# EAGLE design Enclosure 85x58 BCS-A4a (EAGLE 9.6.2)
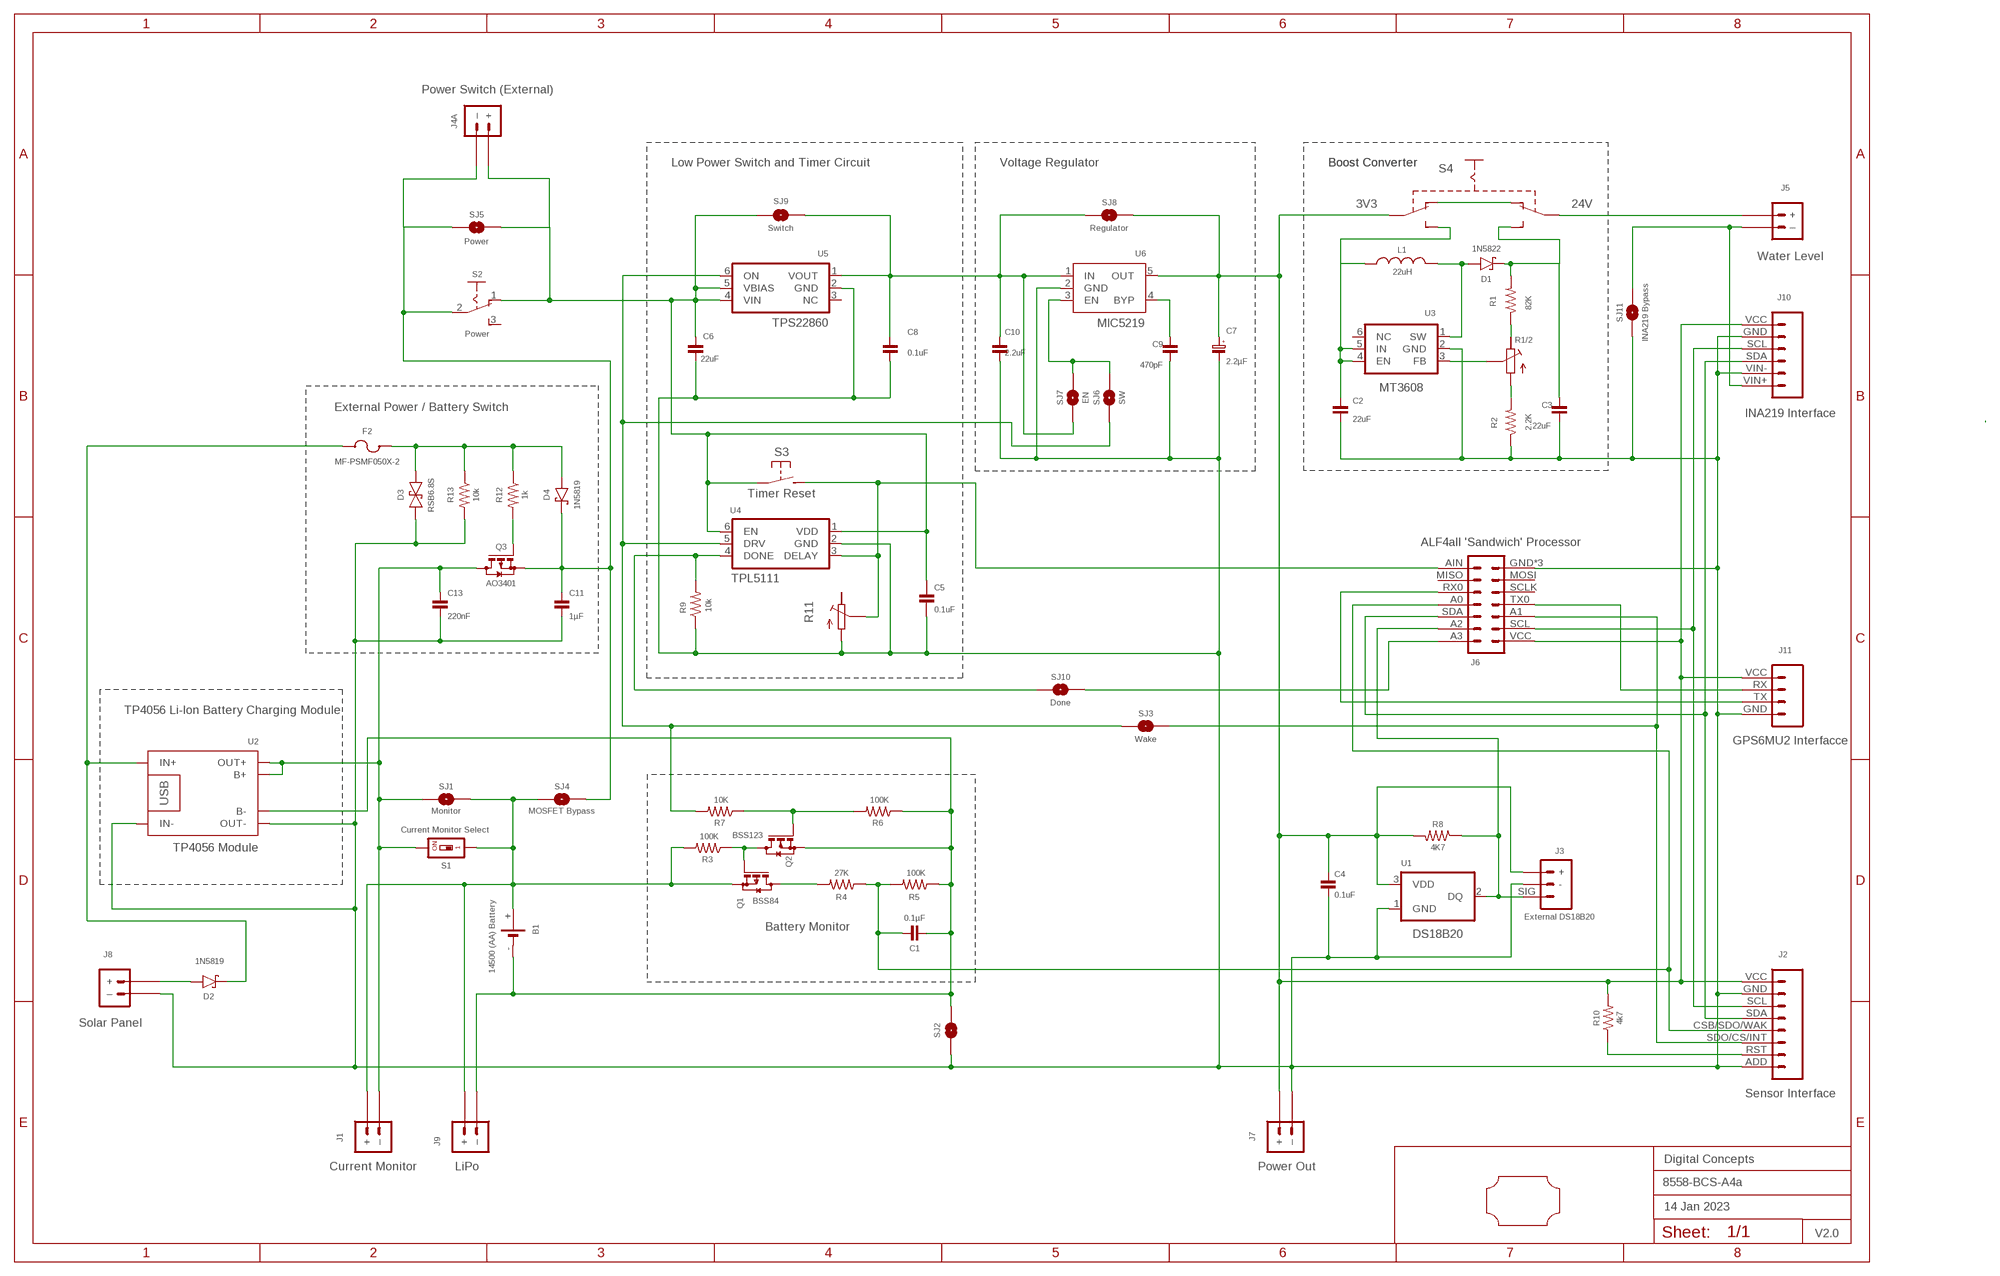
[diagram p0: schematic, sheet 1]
FRAME2 (A3L-LOC): DATE: 14 Jan 2023; OWNER: Digital Concepts; TITLE: 8558-BCS-A4a; VERSION: V2.0

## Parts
B1  14500 (AA) Battery  BATTERY-HOLDER-14500(AA)  [BATTERY-14500]
C1  0.1µF  CAPACITOR-0805  [C0805]
C2  22uF  CAPACITOR-1206  [C1206]
C3  22uF  CAPACITOR-1206  [C1206]
C4  0.1uF  CAPACITOR-0805  [C0805]
C5  0.1uF  CAPACITOR  [C0805@1]
C6  22uF  CAPACITOR-1206  [C1206]
C7  2.2µF  CAPACITOR-1206-TANTALUM  [C1206-POLARISED]
C8  0.1uF  CAPACITOR-0805  [C0805]
C9  470pF  CAPACITOR-0805  [C0805]
C10  2.2uF  CAPACITOR-0805  [C0805]
C11  1µF  CAPACITOR-0805  [C0805]
C13  220nF  CAPACITOR-0805  [C0805]
D1  1N5822  DIODE-SCHOTTKY-1N5822  [DIODE_SMB]
D2  1N5819  1N5819-SOD-123  [SOD-123]
D3  RSB6.8S  DIODE-SCHOTTKY-BIDIRECTIONAL  [VMD2]
D4  1N5819  DIODE-SCHOTTKY-1N5819  [SOD-123]
F2  MF-PSMF050X-2  [F0805]
J1  Current Monitor  JST-PH2.0-2-H-POWER  [JST-PH2.0-2-HORIZONTAL-POWER]
J2  Sensor Interface  HEADER-1X8-SENSOR  [CONN_08-SENSOR]
J3  External DS18B20  JST-PH2.0-3-VERTICAL-SIG  [JST-PH2.0-3-VERTICAL-SIG]
J4A  Power Switch (External)  JST-PH2.0-2-DUAL-POWER"  [JST-PH2.0-2-DUAL-POWER]
J5  Water Level  JST-PH2.0-2-VERTICAL-POWER  [JST-PH2.0-2-VERTICAL-POWER]
J6  ALF4all 'Sandwich' Processor  ALF4ALL-PROCESSOR-BOARD  [ALF4ALL-PROCESSOR-BOARD]
J7  Power Out  JST-GH1.25-2-VERTICAL-POWER  [JST-GH1.25-2-VERTICAL-POWER]
J8  Solar Panel  JST-PH2.0-2-VERTICAL-POWER  [JST-PH2.0-2-VERTICAL-POWER]
J9  LiPo  JST-PH2.0-2-H-POWER  [JST-PH2.0-2-HORIZONTAL-POWER]
J10  INA219 Interface  INA219-I2C-MODULE  [CONN_06-INA219]
J11  GPS6MU2 Interfacce  HEADER-1X4-GPS  [CONN_04-GPS]
L1  22uH  INDUCTOR-CDRH104R/6D28L5038P  [CDRH104R+6D28]
Q1  BSS84  [SOT23]
Q2  BSS123  [SOT23]
Q3  AO3401  MOSFET-AO3401  [SOT-23]
R1  82K  RESISTORR0805  [R0805]
R1/2  RESISTOR-TRIMM-BAOTER-HORIZONTAL  [RTRIM64P]
R2  2.2K  RESISTOR-VIA-1  [R0805-VIA-1]
R3  100K  RESISTORR0805  [R0805]
R4  27K  RESISTORR0805  [R0805]
R5  100K  RESISTORR0805  [R0805]
R6  100K  RESISTORR0805  [R0805]
R7  10K  RESISTORR0805  [R0805]
R8  4K7  RESISTORR0805  [R0805]
R9  10k  RESISTOR-VIA-2  [R0805-VIA-2]
R10  4k7  RESISTORR0805  [R0805]
R11  RESISTOR-TRIMM-BAOTER-HORIZONTAL  [RTRIM64P]
R12  1k  RESISTORR0805  [R0805]
R13  10k  RESISTORR0805  [R0805]
S1  Current Monitor Select  SWITCH-DIP-SWS001-VIA-1  [SMD-001-VIA-1]
S2  Power  SWITCH-SLIDE-SPDT  [SWITCH-SLIDE-SPDT]
S3  Timer Reset  SWITCH-MOMENTARY-2-PIN  [SWITCH-2-PAD]
S4  SWITCH-SLIDE-DPDT-PTH-S  [SWITCH-DPDT-PTH]
SJ1  Monitor  SJ  [SJ]
SJ2  Charge  SJ-V-1  [SJ-VIA-1]
SJ3  Wake  SJ-V-1  [SJ-VIA-1]
SJ4  MOSFET Bypass  SJ  [SJ]
SJ5  Power  SJ-V-1  [SJ-VIA-1]
SJ6  SW  SJ  [SJ]
SJ7  EN  SJ  [SJ]
SJ8  Regulator  SJ  [SJ]
SJ9  Switch  SJ  [SJ]
SJ10  Done  SJ-V-2  [SJ-VIA-2]
SJ11  INA219 Bypass  SJ  [SJ]
U1  DS18B20  [TO-92]
U2  TP4056 Module  BATTERY-CHARGER-LI-PROT  [BATTERY-CHARGER-LI-PROT]
U3  MT3608  [SOT-23-6]
U4  TPL5111  TPL5111DDCR  [SOT-23-6]
U5  TPS22860  [SOT-23-6]
U6  MIC5219  MIC5219XX  [SOT-23-5]
U$1  PCB-OUTLINE-CA-85X58  [PROTO-28X18-OUTLINE-CA]

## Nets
GND: C2.2 C3.2 C4.2 C5.1 C6.2 C7.2(-) C8.1 C9.2 C10.1 C11.2 C13.2 D3.P$2 J2.ADD J2.GND J3.- J6.GND J6.GND@TL J6.GND@TR J7.-(–) J8.-(–) J10.GND J10.VIN- J11.GND R2.1 R2.1@VIA R9.1 R11.1(A) R13.2 SJ2.1 SJ2.1@V SJ11.1 U1.1(GND) U2.IN- U2.OUT- U3.2(GND) U4.2(GND) U5.2(GND) U6.2(GND)
N$1: D2.A J8.+
N$2: C11.1 D4.C J4A.-(–) Q3.2(S) S2.2(P) SJ4.2 SJ5.2
N$3: B1.+ J1.+ J9.+ Q1.2(S) R3.2 S1.1 S1.1@VIA SJ1.2 SJ4.1
N$5: D2.C F2.1 U2.IN+
N$6: D1.A L1.2 U3.1(SW)
N$7: C9.1 U6.4(BYP)
N$8: J2.SCL J6.SCL J10.SCL
N$9: J2.RST R10.1
N$10: C1.1 J2.CSB/SDO/WAK J6.A0 R4.1 R5.2
N$11: J2.SDA J6.SDA J10.SDA
N$13: J3.SIG J6.A2 R8.1 U1.2(DQ)
N$14: J6.TX0 J11.RX
N$15: J5.-(–) J10.VIN+ SJ11.2
N$16: J6.RX0 J11.TX
N$18: C13.1 J1.-(–) Q3.3(D) S1.2 SJ1.1 U2.B+ U2.OUT+
N$19: SJ6.2 SJ7.2 U6.3(EN)
N$20: C8.2 C10.2 SJ7.1 SJ8.1 SJ9.1 U5.1(VOUT) U6.1(IN)
N$22: J6.A3 SJ10.1
N$23: Q1.3(D) R4.2
N$24: C2.1 L1.1 U3.4(EN) U3.5(IN)
N$25: J6.AIN R11.2(S) S3.P$2(S) U4.3(DELAY)
N$27: C5.2 C6.1 J4A.+ S2.1(O) S3.P$1(P) SJ5.1 SJ5.1@V SJ9.2 U4.1(VDD) U4.6(EN) U5.4(VIN) U5.5(VBIAS)
N$28: R7.2 SJ3.2 SJ6.1 U4.5(DRV) U5.6(ON)
N$29: R9.2 R9.2@VIA SJ10.2 SJ10.2@V U4.4(DONE)
N$30: J2.SDO/CS/INT J6.A1 SJ3.1 SJ3.1@V
N$31: C3.1 D1.C R1.2
N$32: R1.1 R1/2.3(E)
N$33: R1/2.2(S) U3.3(FB)
N$34: R1/2.1(A) R2.2
N$35: Q1.1(G) Q2.3(D) R3.1
N$36: S4.P$6(S2)
N$37: Q2.1(G) R6.2 R7.1
N$38: B1.- C1.2 J9.-(–) Q2.2(S) R5.1 R6.1 SJ2.2 U2.B-
N$39: S4.P$1(O1) S4.P$4(O2)
N$41: S4.P$3(S1)
N$42: J5.+ S4.P$5(P2)
N$43: Q3.1(G) R12.2
N$44: D3.P$1 D4.A F2.2 R12.1 R13.1
VCC: C4.1 C7.1(+) J2.VCC J3.+ J6.VCC J7.+ J10.VCC J11.VCC R8.2 R10.2 S4.P$2(P1) SJ8.2 U1.3(VDD) U6.5(OUT)
Unconnected: J6.MISO J6.MOSI J6.SCLK R11.3(E) S2.3(S) U3.6(NC) U5.3(NC)

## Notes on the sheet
- Low Power Switch and Timer Circuit | Voltage Regulator | Boost Converter | Boost Converter
- 3V3 | 24V
- External Power / Battery Switch
- TP4056 Li-Ion Battery Charging Module
- Battery Monitor

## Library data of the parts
B1 = digitalconcepts:BATTERY-HOLDER-14500(AA): 14500 (AA) battery holder
C1 C4 C8-C11 C13 = digitalconcepts:CAPACITOR-0805: 0805 Capacitor
C2 C3 C6 = digitalconcepts:CAPACITOR-1206: 1206 Capacitor
C5 = digitalconcepts:CAPACITOR: 0805 Capacitor
C7 = digitalconcepts:CAPACITOR-1206-TANTALUM: Capacitor 1206 Tantalum
D1 = digitalconcepts:DIODE-SCHOTTKY-1N5822: 1N5822 Schottky Diode SMB
D2 = digitalconcepts:1N5819-SOD-123: 1N5819 Schottky Diode SOD-123
D3 = digitalconcepts:DIODE-SCHOTTKY-BIDIRECTIONAL: Schottky Bidirectional Diode
D4 = digitalconcepts:DIODE-SCHOTTKY-1N5819: 1N5819 Schottky Diode SOD-123
F2 = digitalconcepts:MF-PSMF050X-2: PTC Resettable Fuse
J1 J9 = digitalconcepts:JST-PH2.0-2-H-POWER: JST PH2.0 2P Right Angle Connector with power pin labelling
J2 = digitalconcepts:HEADER-1X8-SENSOR: IoT Sensors 1x8 Pin Header for 'Sandwich' IoT Sensors
J3 = digitalconcepts:JST-PH2.0-3-VERTICAL-SIG: PH2.0 3P Vertical Connector (Sig)
J4A = digitalconcepts:JST-PH2.0-2-DUAL-POWER: PH2.0 2P PTH Dual-Side Connector (Power); PROD_ID: CONN-09863; SKU: PRT-09914
J5 J8 = digitalconcepts:JST-PH2.0-2-VERTICAL-POWER: JST PH2.0 2P PTH Connector (Power)
J6 = digitalconcepts:ALF4ALL-PROCESSOR-BOARD: ALF4all 'Sandwixh' Processor 2x7 Pin Header and earthed 1x1 locator pins for ALF4all 'Sandwich' Processor/RFM95W PCBs
J7 = digitalconcepts:JST-GH1.25-2-VERTICAL-POWER: JST GH1.25 2P PTH Connector (Power)
J10 = digitalconcepts:INA219-I2C-MODULE: INA219 I2C Module
J11 = digitalconcepts:HEADER-1X4-GPS: NEO GPS 4-Pin Header
L1 = digitalconcepts:INDUCTOR-CDRH104R/6D28: Inductor; SPICEPREFIX: L
Q1 = digitalconcepts:BSS84: P-CHANNEL MOS FET
Q2 = digitalconcepts:BSS123: N-CHANNEL MOS FET
Q3 = digitalconcepts:MOSFET-AO3401: AO3401 P-Channel MOSFET
R1 R3-R8 R10 R12 R13 = digitalconcepts:RESISTOR: Resistor; SPICEPREFIX: R
R1/2 R11 = digitalconcepts:RESISTOR-TRIMM-BAOTER-HORIZONTAL: Trimm Resistor - Horizontal BAOTER
R2 = digitalconcepts:RESISTOR-VIA-1: Resistor with via on Pad 1
R9 = digitalconcepts:RESISTOR-VIA-2: Resistor with via on Pad 2
S1 = digitalconcepts:SWITCH-DIP-SWS001-VIA-1: SMD Dip Switch 1 pol.
S2 = digitalconcepts:SWITCH-SLIDE-SPDT: Mini Sliding Switch SPDT
S3 = digitalconcepts:SWITCH-MOMENTARY-2-PIN: 2 Pin Momentary Switch
S4 = digitalconcepts:SWITCH-SLIDE-DPDT-PTH-S: Switch DPDT PTH-S
SJ1 SJ4 SJ6-SJ9 SJ11 = digitalconcepts:SJ: Solder Jumper
SJ2 SJ3 SJ5 = digitalconcepts:SJ-V-1: Solder Jumper with single Pad Via
SJ10 = digitalconcepts:SJ-V-2: Solder Jumper with Pad Vias
U1 = digitalconcepts:DS18B20: Digital Thermometer -55C-125C TO92-3; AVAILABILITY: Bad; DESCRIPTION: Temperature Sensor Digital, Local -55°C ~ 125°C 12 b 8-uMAX; MF: Maxim Integrated; MP: DS18B20; PACKAGE: TO-92 Maxim Integrated; PRICE: None
U2 = digitalconcepts:BATTERY-CHARGER-LI-PROT: TP4056 Li Battery Charger module with PCB (rather than module) footprint
U3 = digitalconcepts:MT3608: MT3608 DC-DC Step-Up Voltage Converter
U4 = digitalconcepts:TPL5111DDCR: TPL5111 Nano-Power System Timer
U5 = digitalconcepts:TPS22860: Texas Instruments TPS22860 Ultra-Low Leakage Load Switch
U6 = digitalconcepts:MIC5219XX: VOLTAGE REGULATOR; OC_FARNELL: unknown; OC_NEWARK: unknown
U$1 = digitalconcepts:PCB-OUTLINE-CA-85X58: PCB outline with cut-out for 85 x 58 enclosure

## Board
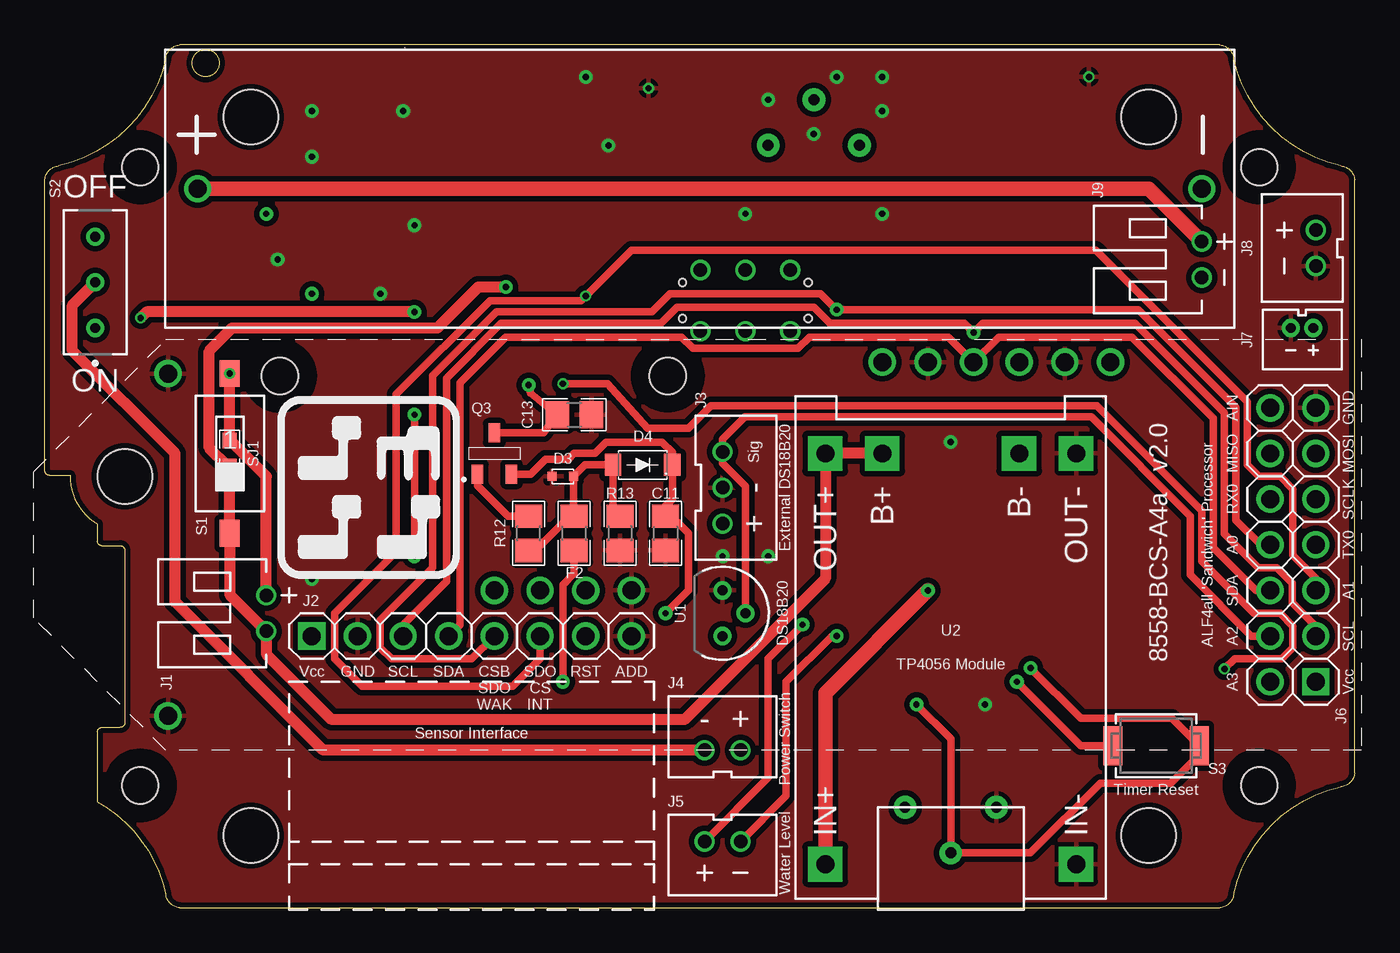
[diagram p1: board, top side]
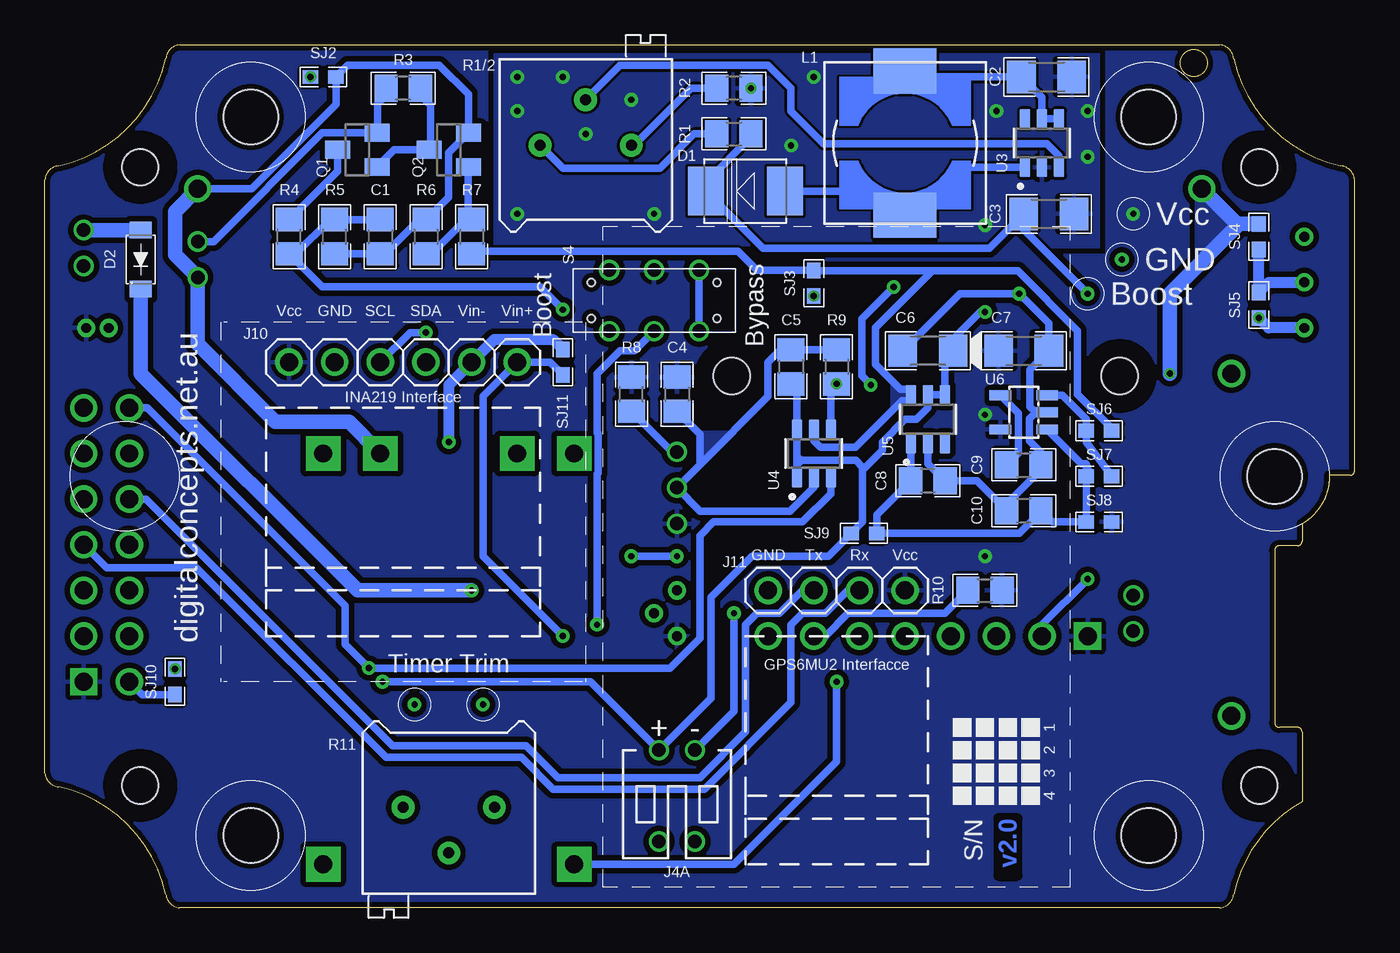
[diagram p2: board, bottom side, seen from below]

Size 72.9 x 48.01 mm. Coordinates in mm from the lower left corner, seen from the top.
Copper layers (1*16): Top 0.035mm / dielectric 1.5mm / Bottom 0.035mm
Design rules "default *": minimum track width 6mil, minimum drill 0.35mm, track to track 6mil, track to pad 6mil, pad to pad 6mil, via to via 6mil, smd to smd 6mil, copper to edge 6mil, drill to drill 6mil, minimum pad ring 1mil, minimum via ring 8mil, stop-mask expansion 4mil, vias tented up to drill 0mil, thermal gap 10mil
Holes 2.03 mm at 13.08,29.59 34.67,29.59

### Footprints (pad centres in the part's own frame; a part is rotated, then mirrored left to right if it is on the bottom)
BATTERY-14500 = drill 1: + -27.94,0; - 27.94,0
C0805 = smd 1.3 x 1.5: 1 -0.95,0; 2 0.95,0
C1206 = smd 1.6 x 1.8: 1 -1.4,0; 2 1.4,0
C0805@1 = smd 1.3 x 1.5: 1 -0.95,0; 2 0.95,0
C1206-POLARISED = smd 1.6 x 1.8: 1 -1.4,0; 2 1.4,0
DIODE_SMB = smd 2 x 2.7: A 2.2,0; C -2.2,0
SOD-123 = smd 0.91 x 1.22: A -1.65,0; C 1.65,0
VMD2 = smd 0.5 x 0.5: P$1 -0.6,0; P$2 0.6,0
F0805 = smd 1.3 x 1.5: 1 -0.95,0; 2 0.95,0
JST-PH2.0-2-HORIZONTAL-POWER = drill 0.75: + 1,0; - -1,0
CONN_08-SENSOR = drill 1 pad 1.524: ADD 17.78,0; CSB/SDO/WAK 10.16,0; GND 2.54,0; RST 15.24,0; SCL 5.08,0; SDA 7.62,0; SDO/CS/INT 12.7,0 | drill 1 pad 1.524 square: VCC 0,0
JST-PH2.0-3-VERTICAL-SIG = drill 0.75: + -2,0; - 0,0; SIG 2,0
JST-PH2.0-2-DUAL-POWER = drill 0.75: + 1,0; - -1,0
JST-PH2.0-2-VERTICAL-POWER = drill 0.75: + -1,0; - 1,0
ALF4ALL-PROCESSOR-BOARD = drill 1 pad 1.524: A0 7.62,2.54; A1 5.08,0; A2 2.54,2.54; A3 0,2.54; AIN 15.24,2.54; GND 15.24,0; GND@TL -1.905,63.881; GND@TR 17.145,63.881; MISO 12.7,2.54; MOSI 12.7,0; RX0 10.16,2.54; SCL 2.54,0; SCLK 10.16,0; SDA 5.08,2.54; TX0 7.62,0 | drill 1 pad 1.524 square: VCC 0,0
JST-GH1.25-2-VERTICAL-POWER = drill 0.55 pad 1.016: + 0.625,0; - -0.625,0
CONN_06-INA219 = drill 1 pad 1.524: GND 2.54,0; SCL 5.08,0; SDA 7.62,0; VCC 0,0; VIN+ 12.7,0; VIN- 10.16,0
CONN_04-GPS = drill 1 pad 1.524: GND 0,0; RX 5.08,0; TX 2.54,0; VCC 7.62,0
CDRH104R+6D28 = smd 2.5 x 3.5: 1 -4,0; 2 4,0
SOT23 = smd 1 x 1.4: 1 -0.95,-1.1; 2 0.95,-1.1; 3 0,1.1
SOT-23 = smd 0.65 x 1.05: 1 -0.95,-1.15; 2 0.95,-1.15; 3 0,1.15
R0805 = smd 1.3 x 1.5: 1 -0.95,0; 2 0.95,0
RTRIM64P = drill 0.61 pad 1.27: 1 0,-2.54; 2 2.54,0; 3 0,2.54
R0805-VIA-1 = smd 1.3 x 1.5: 1 -0.95,0; 2 0.95,0 | drill 0.35 pad 0.61: 1@VIA -0.95,0
R0805-VIA-2 = smd 1.3 x 1.5: 1 -0.95,0; 2 0.95,0 | drill 0.35 pad 0.61: 2@VIA 0.95,0
SMD-001-VIA-1 = smd 1.1 x 1.5: 1 0,-4.45; 2 0,4.45 | drill 0.35 pad 0.61: 1@VIA 0,-4.45
SWITCH-SLIDE-SPDT = drill 0.55 pad 1.016: 1 -2.54,0; 2 0,0; 3 2.54,0
SWITCH-2-PAD = smd 1.067 x 2.184: P$1 -2.4,0; P$2 2.4,0
SWITCH-DPDT-PTH = drill 0.75: P$1 -1.7,2.5; P$2 -1.7,0; P$3 -1.7,-2.5; P$4 1.7,2.5; P$5 1.7,0; P$6 1.7,-2.5 | hole 0.42: 1,3.5; -1,3.5; 1,-3.5; -1,-3.5
SJ = smd 0.864 x 0.762: 1 -0.711,0; 2 0.711,0
SJ-VIA-1 = smd 0.864 x 0.762: 1 -0.711,0; 2 0.711,0 | drill 0.35 pad 0.61: 1@V -0.711,0
SJ-VIA-2 = smd 0.864 x 0.762: 1 -0.711,0; 2 0.711,0 | drill 0.35 pad 0.61: 2@V 0.711,0
TO-92 = drill 0.55 pad 1.016: 1 -1.27,0; 2 0,1.27; 3 1.27,0
BATTERY-CHARGER-LI-PROT = drill 1 pad 1.93 square: B+ 10.795,3.81; B- 10.795,-3.81; IN+ -12.065,6.985; IN- -12.065,-6.985; OUT+ 10.795,6.985; OUT- 10.795,-6.985
SOT-23-6 = smd 1.1 x 0.6: 1 -1.35,0.95; 2 -1.35,0; 3 -1.35,-0.95; 4 1.35,-0.95; 5 1.35,0; 6 1.35,0.95
SOT-23-5 = smd 0.55 x 1.2: 1 -0.95,-1.3; 2 0,-1.3; 3 0.95,-1.3; 4 0.95,1.3; 5 -0.95,1.3
PROTO-28X18-OUTLINE-CA = hole 2.032: -31.14,17.196; -31.14,-17.196; 31.14,-17.196; 31.14,17.196 | hole 3.048: -24.994,19.99; -32.004,0; -24.994,-19.99; 24.994,-19.99; 24.994,19.99

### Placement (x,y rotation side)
B1  36.45,40.01 0 top
C1  54.23,37.34 270 bottom
C2  17.14,46.23 0 bottom
C3  17.02,38.61 0 bottom
C4  37.72,28.58 270 bottom
C5  31.37,30.1 270 bottom
C6  23.75,30.99 180 bottom
C7  18.41,30.99 0 bottom
C8  23.75,23.75 180 bottom
C9  18.41,24.64 0 bottom
C10  18.41,22.1 0 bottom
C11  34.54,20.83 270 top
C13  29.46,27.43 0 top
D1  33.91,39.88 0 bottom
D2  67.56,36.07 270 bottom
D3  28.83,24 180 top
D4  33.27,24.64 0 top
F2  29.46,20.83 90 top
J1  12.32,16.38 90 top
J2  14.86,15.11 0 top
J3  37.72,23.37 90 top
J4A  37.72,8.76 180 bottom
J5  37.72,3.68 0 top
J6  70.74,12.57 90 top
J7  69.98,32.26 0 top
J8  70.74,36.7 270 top
J9  64.39,36.07 90 top
J10  59.31,30.35 0 bottom
J11  32.64,17.65 0 bottom
L1  25.02,42.55 270 bottom
Q1  55.5,42.16 90 bottom
Q2  50.42,42.16 90 bottom
Q3  25.02,25.27 0 top
R1  34.54,43.05 0 bottom
R1/2  42.8,42.42 90 bottom
R2  34.54,45.59 180 bottom
R3  52.96,45.59 180 bottom
R4  59.31,37.34 90 bottom
R5  56.77,37.34 90 bottom
R6  51.69,37.34 270 bottom
R7  49.15,37.34 270 bottom
R8  40.26,28.58 90 bottom
R9  28.83,30.1 270 bottom
R10  20.57,17.65 0 bottom
R11  50.42,5.59 270 bottom
R12  26.92,20.83 90 top
R13  32,20.83 270 top
S1  10.29,25.27 180 top
S2  2.79,34.8 90 top
S3  61.85,9.02 0 top
S4  38.99,33.78 270 bottom
SJ1  10.29,25.27 90 top
SJ2  57.4,46.23 0 bottom
SJ3  30.1,34.75 90 bottom
SJ4  5.33,37.34 270 bottom
SJ5  5.33,33.53 90 bottom
SJ6  14.22,26.54 180 bottom
SJ7  14.22,24 0 bottom
SJ8  14.22,21.46 0 bottom
SJ9  27.3,20.83 180 bottom
SJ10  65.66,12.57 90 bottom
SJ11  44.07,30.35 270 bottom
U1  37.72,16.38 270 top
U2  50.42,14.48 90 top
U3  17.4,42.55 90 bottom
U4  30.1,25.27 90 bottom
U5  23.75,27.18 90 bottom
U6  18.41,27.56 90 bottom
U$1  36.45,24 0 top

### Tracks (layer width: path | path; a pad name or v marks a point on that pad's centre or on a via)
$X1
  cutout Bottom: 67.59,43.23 arc180 67.59,39.17 arc180
$X2
  cutout Bottom: 67.59,8.84 arc180 67.59,4.78 arc180
$X3
  cutout Bottom: 5.31,8.84 arc180 5.31,4.78 arc180
$X4
  cutout Top: 5.31,43.23 arc180 5.31,39.17 arc180
$X5
  cutout Bottom: 5.31,43.23 arc180 5.31,39.17 arc180
$X6
  cutout Top: 67.59,43.23 arc180 67.59,39.17 arc180
$X7
  cutout Top: 67.59,8.84 arc180 67.59,4.78 arc180
$X8
  cutout Top: 5.31,8.84 arc180 5.31,4.78 arc180
$X9
  cutout Bottom: 13.08,31.62 arc180 13.08,27.56 arc180
$X10
  cutout Top: 13.08,31.62 arc180 13.08,27.56 arc180
$X11
  cutout Bottom: 34.67,31.62 arc180 34.67,27.56 arc180
GND  (via drill 0.35)
  Bottom 0.406: R9.1 C5.1 31.94,31.05 32.64,30.35 32.64,28.45 36.45,24.64 | U4.2 30.1,23.4 31.43,22.07 36.42,22.07 J3.- 36.45,24.64 | 17.75,27.56 18.1,27.2 18.1,25.98 17.46,25.34 C9.2 17.46,24.38 19.36,22.48 C10.1 21.02,23.75 C8.1 23.69,24.64 23.69,24.65 23.75,24.7 U5.2 | U6.2 17.75,27.56 | C4.2 36.45,26.36 36.45,24.64 | 17.75,27.56 18.07,27.88 18.07,29.93 C7.2 17.01,32.51 v18.67,34.16 21.97,34.16 C6.2 | v14.86,18.29 17.4,15.75 J2.GND | v37.72,19.56 v40.26,19.56
  Bottom 0.61: SJ11.1 44.63,31.62 47.88,31.62 J10.VIN- 50.42,29.08 v50.42,25.91
  other vias: 46.61,38.61 14.86,41.78 30.1,46.23 20.57,37.97 46.61,44.32 46.61,46.23 12.95,36.07 52.32,11.3 14.86,44.32 19.94,44.32 31.37,42.42 38.99,38.61 44.07,46.23 40.26,44.96 42.8,43.05
  pour Top (isolate 0.305): -2.08,49.93 -2.08,-1.97 74.92,-1.97 74.92,49.93
  pour Bottom: 47.88,47.5 47.88,36.92 14.22,36.73 14.22,47.5
  pour Bottom: 36.45,24.64 36.45,26.36 34.74,26.36
N$1
  Bottom 0.813: D2.A 67.58,37.7 J8.+
N$2  (via drill 0.35)
  Top 0.406: Q3.2 27.04,24.12 27.88,24.96 29.15,24.96 29.46,25.27 30.61,25.27 31.24,25.91 34.35,25.91 34.92,25.34 D4.C 34.92,22.73 34.54,22.35 C11.1 34.86,21.78 35.81,20.83 35.81,17.65 v34.54,16.38
  Top 0.61: S2.2 1.52,33.53 1.52,30.99 7.24,25.27 7.24,17.02 15.49,8.76 J4A.-
  Bottom 0.406: J4A.- 34.54,10.94 v34.54,16.38
  Bottom 0.61: S2.2 4.77,34.8 SJ5.2 SJ4.2
N$3
  Top 0.61: J1.+ 12.32,24 10.34,25.98 SJ1.2 S1.1
  Top 0.813: J9.+ 61.45,40.01 B1.+
  Bottom 0.406: R3.2 53.91,45.19 54.37,44.73 54.37,43.15 Q1.2 57.47,43.11 63.52,37.07 J9.+
  Bottom 0.813: S1.1 10.29,34.17 6.4,38.05 SJ4.1 6.6,38.05 6.58,38.08 B1.+
  pour Bottom: 8.51,39.88 6.6,37.97 8.51,36.07
N$5  (via drill 0.35)
  Top 0.406: F2.1 29.46,18.61 28.83,17.97 v28.83,12.57
  Top 0.813: U2.IN+ 43.43,11.94 v49.15,17.65
  Bottom 0.406: v28.83,12.57 28.83,8.13 34.54,2.41 U2.IN+
  Bottom 0.813: D2.C 67.56,29.72 55.5,17.65 v49.15,17.65
N$6
  Bottom 0.406: D1.A 26.99,39.88 25.65,38.55 L1.2 24.38,38.55 21.73,41.2 U3.1
N$7
  Bottom 0.406: U6.4 18.72,27.52 18.72,25.28 C9.1
N$8  (via drill 0.35)
  Top 0.406: J6.SCL 70.74,15.67 69.44,16.97 69.44,18.06 68.58,18.92 67.54,18.92 65.66,20.8 65.66,27.53 60.68,32.51 52.2,32.51 v51.69,32 51.18,32.51 43.69,32.51 42.8,33.4 35.18,33.4 34.29,32.51 25.4,32.51 22.35,29.46 22.35,18.16 19.94,15.75 J2.SCL
  Bottom 0.406: v51.69,32 52.58,32 J10.SCL
N$9
  Bottom 0.406: J2.RST 29.46,15.11 28.19,16.38 22.79,16.38 R10.1
N$10  (via drill 0.35)
  Top 0.406: J2.CSB/SDO/WAK 23.75,13.84 19.3,13.84 18.67,14.48 18.67,16 21.59,18.92 21.59,29.59 25.15,33.15 33.78,33.15 34.8,34.16 43.18,34.16 v44.07,33.27 60.86,33.27 66.29,27.84 66.29,21.57 67.67,20.19 J6.A0
  Bottom 0.406: v44.07,33.27 45.34,34.54 57.47,34.54 R4.1 58.93,36.39 57.03,38.29 R5.2 C1.1
N$11
  Top 0.406: J6.SDA 67.41,17.65 65.02,20.04 65.02,27.23 60.5,31.75 53.09,31.75 J10.SDA 50.29,31.75 42.54,31.75 41.91,31.12 36.07,31.12 35.43,31.75 25.65,31.75 23.11,29.21 23.11,15.75 J2.SDA
N$13
  Top 0.406: J6.A2 67.16,15.11 63.75,18.52 63.75,21.79 58.24,27.3 38.96,27.3 37.72,26.07 J3.SIG 37.72,24.73 38.99,23.46 U1.2
  Bottom 0.406: J3.SIG 38,25.37 R8.1
N$14
  Bottom 0.406: J11.RX 28.19,17.65 29.46,16.38 30.73,16.38 31.37,15.75 31.37,11.43 36.2,6.6 44.6,6.6 46.38,8.38 53.9,8.38 64.48,18.92 69.47,18.92 J6.TX0
N$15  (via drill 0.35)
  Top 0.406: v44.07,15.11 43.8,15.11 41.26,12.57 41.26,6.22 J5.-
  Bottom 0.406: SJ11.2 44.78,30.35 J10.VIN+ 48.51,28.45 48.51,19.56 v44.07,15.11
N$16
  Bottom 0.406: J6.RX0 67.26,22.73 53.54,9.02 46.13,9.02 44.35,7.24 36.45,7.24 33.91,9.78 33.91,15.75 33.27,16.38 32,16.38 30.73,17.65 J11.TX
N$18  (via drill 0.35)
  Top 0.406: Q3.3 27.76,26.42 C13.1 27.03,28.62 v26.92,29.08
  Top 0.61: U2.B+ U2.OUT+ 43.43,18.31 35.59,10.47 15.97,10.47 12.32,14.11 J1.- 10.29,17.41 S1.2 SJ1.1 10.16,24.56 9.14,25.58 9.14,30.99 10.41,32.26 21.84,32.26 24.13,34.54 v25.65,34.54
  Bottom 0.406: v26.92,29.08 27.43,29.59 27.43,32.77 v25.65,34.54
N$19
  Bottom 0.406: SJ7.2 14.93,25.91 SJ6.2 14.93,27.18 16.27,28.51 U6.3
N$20
  Bottom 0.406: U6.1 15.21,24.7 14.96,24.7 | SJ7.1 14.74,24.2 14.96,24.7 | 14.96,24.7 14.93,24.67 SJ8.1 16.83,21.46 C10.2 17.46,22.03 18.67,20.83 SJ9.1 26.59,21.85 C8.2 U5.1
N$22
  Bottom 0.406: J6.A3 67.49,11.86 SJ10.1
N$23
  Bottom 0.406: Q1.3 56.62,41.77 56.62,40.98 R4.2
N$24
  Bottom 0.406: U3.4 U3.5 17.4,45.08 C2.1 | L1.1 24.7,46.23 C2.1 | C2.1
N$25  (via drill 0.35)
  Top 0.406: v54.86,13.34 57.66,10.54 62.72,10.54 S3.P$2 64.25,8.51 62.67,6.93 58.75,6.93 54.86,3.05 R11.2 50.42,9.4 v48.51,11.3
  Bottom 0.406: U4.3 29.15,23.03 30.72,21.46 35.69,21.46 36.45,20.7 36.45,14.99 38.1,13.34 v54.86,13.34 56.19,14.66 56.19,16.79 67.21,27.81 J6.AIN
N$26
  pour Bottom: 27.3,24.43 27.76,24.89 26.85,24.89
N$27  (via drill 0.35)
  Top 0.406: S3.P$1 57.66,9.02 v54.1,12.57
  Top 0.61: v20.57,33.15 5.66,33.15 SJ5.1@V
  Bottom 0.406: 31.05,25.15 U4.6 31.05,28.83 C5.2 | 31.05,25.15 U4.1 31.05,24.64 30.89,24.8 | 30.89,24.8 30.79,24.89 27.76,24.89 27.38,24.51 | v54.1,12.57 42.53,12.57 J4A.+ 35.81,11.67 35.81,17.27 33.53,19.56 29.29,19.56 SJ9.2 27.38,21.46 27.38,24.51 | 27.38,24.51 27.3,24.44 26.29,25.45 26.29,25.91 25.02,27.18 24.38,27.18 23.75,27.81 U5.5 U5.4 22.8,30.54 C6.1 22.35,31.62 20.82,33.15 v20.57,33.15 | 30.89,24.8 30.89,24.99 31.05,25.15
  Bottom 0.61: SJ5.1@V 4.77,32.26 S2.1
N$28
  Bottom 0.406: U4.5 30.1,25.99 29.74,25.63 27.77,25.63 25.21,28.2 24.7,28.2 U5.6 24.7,28.86 25.28,28.86 26.67,30.25 26.67,32.26 23.49,35.43 | R7.2 49.02,36.52 34.33,36.52 33.27,35.46 SJ3.2 30.1,35.43 23.49,35.43 | SJ6.1 13.51,26.67 15.42,28.58 15.42,32.11 18.74,35.43 23.49,35.43
  pour Bottom: 24.93,28.49 25.65,29.21 25.65,27.76
N$29
  Top 0.406: R9.2@VIA 31.3,29.15 33.53,26.67 35.81,26.67 37.08,27.94 58.55,27.94 64.39,22.1 64.39,19.28 67.28,16.38 68.76,16.38 69.47,15.67 69.47,14.45 68.86,13.84 66.22,13.84 SJ10.2@V
  Bottom 0.406: R9.2@VIA 29.15,28.83 U4.4
N$30
  Top 0.406: J6.A1 70.74,18.34 69.47,19.61 69.47,23.29 68.76,24 67.56,24 66.93,24.64 66.93,28.14 58.5,36.58 32.64,36.58 SJ3.1@V 29.84,33.78 24.76,33.78 19.56,28.58 19.56,19.81 16.13,16.38 16.13,13.84 17.65,12.32 26.03,12.32 27.56,13.84 J2.SDO/CS/INT
N$31  (via drill 0.35)
  Bottom 0.406: R1.2 33.59,42.89 36.11,40.38 D1.C 32.93,36.7 20.32,36.7 C3.1 18.42,37.72 v14.86,34.16
N$32
  Bottom 0.406: R1/2.3 44.07,41.15 38.67,41.15 36.76,43.05 R1.1
N$33
  Bottom 0.406: R1/2.2 40.89,46.86 32.64,46.86 31.37,45.59 31.37,44.32 29.55,42.5 17.12,42.5 16.45,41.83 U3.3
N$34
  Bottom 0.406: R2.2 36.93,45.59 40.1,42.42 R1/2.1
N$35
  Bottom 0.406: R3.1 52.01,45.21 51.44,44.65 51.44,42.24 Q2.3 53.45,42.16 Q1.1
N$37
  Bottom 0.406: R6.2 51.37,36.39 49.47,38.29 R7.1 49.35,38.49 49.35,41.18 Q2.1
N$38
  Bottom 0.406: B1.- 61.39,40.01 56.69,44.7 SJ2.2 56.06,46.86 50.95,46.86 49.32,45.25 Q2.2 50.43,42 50.43,39.54 R6.1 52.07,38.29 53.97,36.39 C1.2 R5.1
  Bottom 0.813: U2.B- 55.97,27.05 60.07,27.05 64.39,31.37 J9.- 65.66,36.34 65.66,38.73 B1.-
N$39
  Bottom 0.406: S4.P$1 S4.P$4
N$42  (via drill 0.35)
  Top 0.406: J5.+ 40.26,7.22 40.26,13.84 v42.16,15.75
  Bottom 0.406: S4.P$5 40.08,30.99 40.89,30.99 42.16,29.72 42.16,26.44 42.11,26.39 42.11,24.16 42.16,24.11 v42.16,15.75
N$43
  Top 0.406: R12.2 25.78,21.78 24.07,23.49 Q3.1
N$44
  Top 0.406: R12.1 27.3,19.88 28.95,21.52 29.2,21.52 F2.2 29.43,21.78 D3.P$1 30.06,24.64 D4.A 31.62,22.16 R13.1
VCC  (via drill 0.35)
  Top 0.406: v20.57,27.43 v20.57,19.56
  other vias: 12.32,38.61
  pour Bottom (isolate 0.305, rank 2): -1.08,48.93 -1.08,-0.97 73.92,-0.97 73.92,48.93
X$1
  cutout Bottom: 13.08,31.62 arc-180 13.08,27.56 arc-180
X$2
  cutout Top: 13.08,31.62 arc-180 13.08,27.56 arc-180
X$3
  cutout Top: 34.67,31.62 arc-180 34.67,27.56 arc-180
X$4
  cutout Bottom: 34.67,31.62 arc-180 34.67,27.56 arc-180

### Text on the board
Bottom: v2.0
tPlace: OFF | ON | AIN | GND | MISO | MOSI | RX0 | SCLK | 8558-BCS-A4a v2.0 | A0 | TX0 | SDA | A1 | A2 | SCL | Vcc | GND | SCL | SDA | RST | ADD | A3 | Vcc | CSB / SDO / WAK | SDO / CS / INT
bPlace: Vcc | GND | Boost | Vin+ | Vin- | SDA | SCL | GND | Vcc | digitalconcepts.net.au | Vcc | Rx | Tx | GND | Timer Trim | 1 | 2 | 3 | 4 | S/N
tNames: TP4056 Module | J4 | Power Switch
bNames: Bypass | Boost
